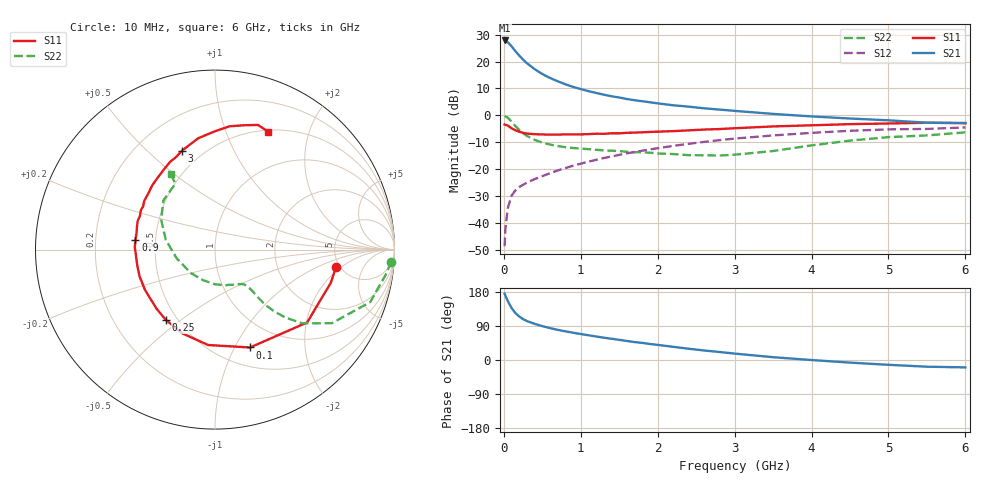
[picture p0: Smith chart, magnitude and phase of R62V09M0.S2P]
! SIEMENS Small Signal Semiconductors
! BFR193
! Si NPN RF Bipolar Junction Transistor in SOT23
! VCE = 2 V  IC = 9 mA
! Common Emitter S-Parameters:  May  1996
# GHz  S  MA  R  50
!  f  S11  S21  S12  S22
! GHz  MAG  ANG  MAG  ANG  MAG  ANG  MAG  ANG
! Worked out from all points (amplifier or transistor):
!   36 points, 10 MHz to 6 GHz, reference 50 ohm
!   highest |S21| = 27.8 dB at 10 MHz (marker M1)
!   |S21| within 3 dB of that: start of sweep to 123.6 MHz
!   unconditionally stable (mu >= 1): 740.9 MHz to 2.004 GHz
!   at 250 MHz: K = 0.62, MSG = 23.2 dB, |S12| = -25.7 dB
!   at 1.4 GHz: K = 1.04, MAG = 9.9 dB, |S12| = -15.2 dB
!   at 6 GHz: K = 0.96, MSG = 0.8 dB, |S12| = -4.4 dB
!   S11 on the Smith chart (normalised r, x): 10 MHz: 4.62, -1.69; 100 MHz: 0.70, -1.15; 250 MHz: 0.43, -0.44; 900 MHz: 0.38, +0.05; 3 GHz: 0.39, +0.65; 6 GHz: 0.52, +1.42
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0.01  0.681 -8.3  24.53 175.1  0.0038 85.3  0.9833 -4.0
0.02  0.6711 -16.0  24.4 169.8  0.0079 83.5  0.9644 -7.9
0.05  0.6545 -38.3  22.89 156.0  0.0189 72.9  0.9128 -18.7
0.1  0.5793 -70.3  19.17 137.3  0.0326 62.6  0.7694 -32.2
0.15  0.533 -94.1  15.56 123.8  0.0411 56.7  0.6368 -40.2
0.2  0.5008 -111.3  12.88 114.9  0.0472 54.2  0.5427 -44.1
0.25  0.478 -125.0  10.83 107.8  0.0521 53.6  0.469 -46.4
0.3  0.4627 -134.9  9.301 102.8  0.0571 54.1  0.4196 -47.6
0.4  0.4502 -150.0  7.22 95.5  0.0663 55.6  0.3545 -48.1
0.5  0.446 -160.4  5.857 89.3  0.0751 57.2  0.314 -47.9
0.6  0.4419 -168.7  4.962 84.2  0.0853 59.1  0.2889 -48.2
0.7  0.4418 -176.1  4.303 79.6  0.0958 60.2  0.2724 -48.8
0.9  0.4467 173.2  3.382 72.0  0.1175 61.1  0.2505 -50.4
1.1  0.4524 164.1  2.831 65.3  0.1394 61.6  0.2383 -54.2
1.3  0.4583 156.0  2.429 58.9  0.1631 60.9  0.2259 -58.3
1.6  0.4781 145.7  2.018 50.2  0.1991 59.3  0.2124 -67.1
2.2  0.5133 128.2  1.547 34.8  0.2734 53.7  0.193 -90.0
3  0.5809 108.5  1.218 16.9  0.3736 42.9  0.1879 -136.8
3.5  0.6273 98.6  1.071 7.4  0.4274 35.2  0.2198 -167.6
4.5  0.6916 83.3  0.879 -6.9  0.5213 20.0  0.3429 151.0
5.5  0.7347 71.0  0.736 -17.7  0.5639 4.5  0.4277 121.1
6  0.7206 65.6  0.726 -19.5  0.6013 -0.1  0.4874 120.3
